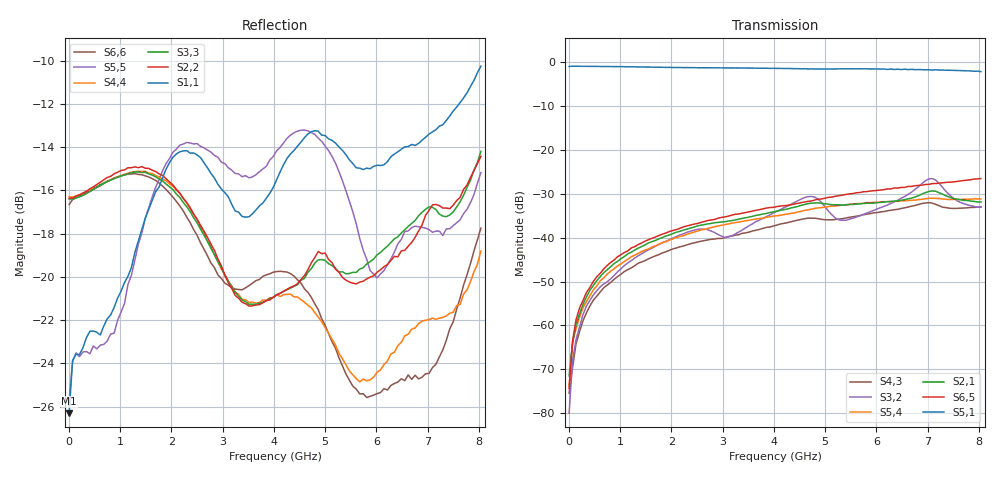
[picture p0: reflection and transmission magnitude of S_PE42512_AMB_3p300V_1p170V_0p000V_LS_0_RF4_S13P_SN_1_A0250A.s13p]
! Device ID: PE42512
! File Path: z:\PE42512\TE_GND_Post_Char_S-Param\All Parts\AMB\3p300\LS_0_RF4\PE42512_AMB_3p300V_1p170V_0p000V_LS_0_RF4_S13P_SN_1_A0250A.s13p
! Serial: 1
! Lot: A0250A
! Temp: AMB
! VDD: 3.300
! VSS: 0.000
! Control_Hi: 1.170
! Control_Lo: 0.000
! Logic State: LS_0_RF4
! Port 1:
! Port 2:
! Port 3:
! Port 4:
! Port 5:
! Port 6:
! Port 7:
! Port 8:
! Port 9:
! Port 10:
! Port 11:
! Port 12:
! Port 13:
! ThroughPath:1-5
! IDD: 0.0001072401
! ISS/IDD2: -2.38e-008
! IDMM3/IDD3: -2.281e-007
! Comment:
#  Hz  S  RI  R  50
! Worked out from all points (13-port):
!   120 points, 10 MHz to 8.037 GHz, reference 50 ohm
!   strongest paths, dB at 10 MHz, 2.034 GHz, 4.057 GHz, 6.08 GHz, 8.037 GHz:
!     S5,1: -1.0, -1.2, -1.4, -1.6, -2.2
!     S6,5: -74.3, -38.4, -32.9, -29.1, -26.5
!     S2,1: -71.5, -39.0, -33.9, -32.0, -31.9
!     S5,4: -73.8, -40.3, -35.0, -31.9, -31.2
!     S3,2: -80.0, -40.1, -34.0, -33.1, -33.0
!     S4,3: -75.4, -42.5, -37.1, -34.1, -33.0
!   lowest |S11| = -26.3 dB at 10 MHz (marker M1), VSWR 1.10, Z = 54.1 - j2.97 ohm
!   |S11| at or under -10 dB: start of sweep to end of sweep
